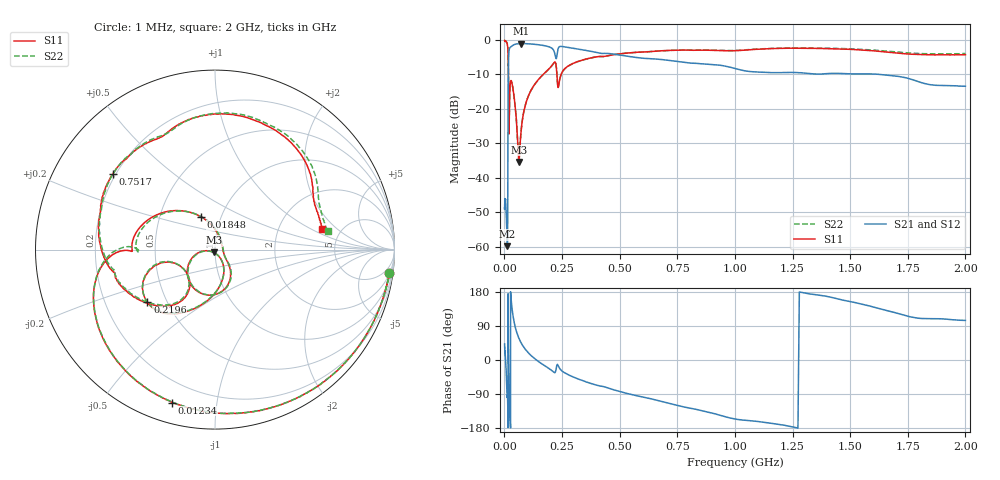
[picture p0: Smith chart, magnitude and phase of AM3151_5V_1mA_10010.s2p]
! Date/Time: Fri Jun 26 10:55:15 2020
! Network Analyzer:  Rev:
! Sweep from 1000000.0 to 2000000000.0, 1601 Points ! Power Supply: 0 V, 0 A
# HZ S DB R 50
!freq MagS11 AngS11 MagS21 AngS21 MagS12 AngS12 MagS22 AngS22
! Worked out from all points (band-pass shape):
!   1601 points, 1 MHz to 2 GHz, reference 50 ohm
!   highest |S21| = -1.05 dB at 72.6 MHz (marker M1); lowest = -59.9 dB at 13.38 MHz (marker M2)
!   |S21| within 3 dB of the highest: 19.16 MHz to 219 MHz (199.8 MHz wide, 168 % of centre); 229.1 MHz to 465.9 MHz (236.7 MHz wide, 68.1 % of centre)
!   lowest |S11| = -35.4 dB at 63.26 MHz (marker M3), VSWR 1.03, Z = 49.3 - j1.52 ohm
!   |S11| at or under -10 dB: 17.93 MHz to 169 MHz (151 MHz wide, 162 % of centre); 227.9 MHz to 246.2 MHz (18.29 MHz wide, 7.72 % of centre)
!   |S22| runs from -35.1 to -0.2 dB; largest |S21 - S12| = 0.0067
!   S11 on the Smith chart (normalised r, x): 1 MHz: 2, -14; 12.34 MHz: 0.10, -0.75; 18.48 MHz: 0.80, +0.31; 219.6 MHz: 0.39, -0.30; 751.7 MHz: 0.19, +0.32; 2 GHz: 3.59, +1.34
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1000000  -0.17 -7.8  -48.71 42.3  -49.16 39.1  -0.17 -7.8
3555161  -0.28 -26.6  -46.08 14.8  -46.07 14.4  -0.27 -26.7
7353941  -0.47 -56.4  -49.27 -21.6  -49.23 -21.1  -0.46 -56.6
1.234248e7  -1.06 -105.7  -58.41 -99.0  -58.47 -97.4  -1.11 -106.4
1.263916e7  -1.14 -109.6  -58.89 -95.9  -58.90 -96.0  -1.17 -110.3
1.338062e7  -1.37 -119.8  -59.87 -94.1  -59.71 -92.2  -1.39 -120.7
1.43689e7  -1.79 -136.2  -52.57 -107.8  -52.61 -107.0  -1.87 -137.6
1.649128e7  -6.68 -178.8  -12.35 123.4  -12.35 123.4  -7.50 -178.6
1.848288e7  -14.03 113.2  -5.11 -7.7  -5.10 -7.7  -14.27 111.2
1.984801e7  -27.17 19.2  -3.44 -60.4  -3.43 -60.4  -26.86 14.5
2.121295e7  -21.81 -40.8  -2.78 -97.3  -2.78 -97.3  -21.87 -40.2
2.614444e7  -12.39 -83.0  -2.12 -172.7  -2.11 -172.7  -12.44 -81.2
4.493426e7  -18.14 -163.0  -1.32 92.5  -1.32 92.4  -18.20 -161.7
6.325922e7  -35.43 -114.3  -1.10 56.9  -1.09 57.0  -35.12 -111.3
7.260301e7  -26.46 -59.1  -1.05 45.2  -1.07 45.1  -26.33 -59.0
1.589914e8  -10.67 -99.4  -1.51 -8.6  -1.51 -8.8  -10.70 -99.8
2.196176e8  -6.41 -142.1  -4.24 -33.2  -4.22 -33.1  -6.42 -142.5
2.369614e8  -12.62 -126.9  -2.07 -19.5  -2.07 -19.4  -12.62 -128.3
5.652395e8  -3.66 170.7  -5.05 -93.1  -5.01 -93.0  -3.64 168.7
7.516596e8  -2.99 143.5  -6.24 -119.9  -6.25 -119.7  -2.99 141.1
1.273592e9  -2.39 82.0  -9.52 -179.6  -9.44 -179.8  -2.31 79.4
2e9  -4.29 11.0  -13.44 104.5  -13.55 103.8  -3.94 9.3
